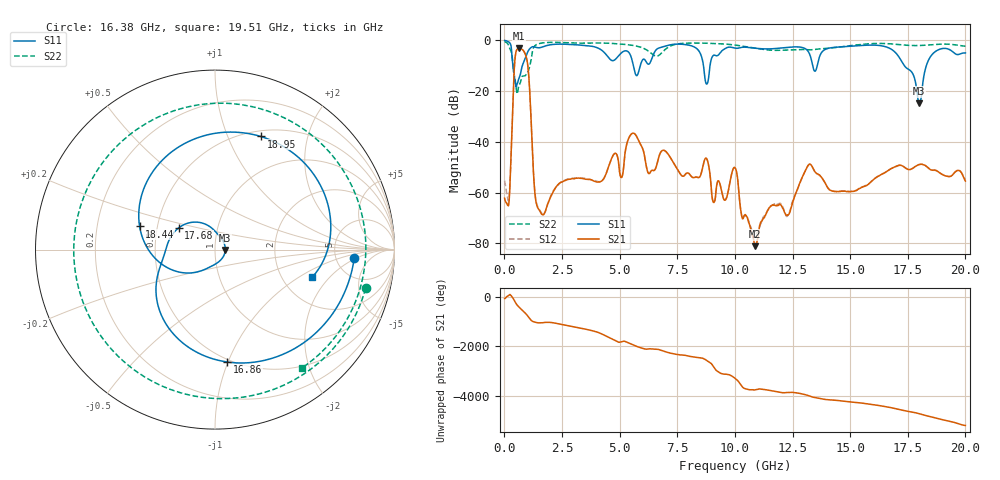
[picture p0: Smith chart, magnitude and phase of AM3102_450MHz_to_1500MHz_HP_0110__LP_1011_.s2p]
!Agilent Technologies,E8364B,MY43040894,A.07.50.67
!Agilent E8364B: A.07.50.67
!Date: Thursday, January 11, 2018 05:49:09
!Correction: S11(Full 2 Port(1,2))
!S21(Full 2 Port(1,2))
!S12(Full 2 Port(1,2))
!S22(Full 2 Port(1,2))
!S2P File: Measurements: S11, S21, S12, S22:
# Hz S  dB  R 50
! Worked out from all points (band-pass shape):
!   1601 points, 10 MHz to 20 GHz, reference 50 ohm
!   highest |S21| = -3.21 dB at 634.7 MHz (marker M1); lowest = -81.1 dB at 10.87 GHz (marker M2)
!   |S21| within 3 dB of the highest: 473.6 MHz to 934.7 MHz (461.1 MHz wide, 65.5 % of centre)
!   lowest |S11| = -24.8 dB at 18 GHz (marker M3), VSWR 1.12, Z = 56.1 - j0.257 ohm
!   |S11| at or under -10 dB: 370 MHz to 778.3 MHz (408.3 MHz wide, 71.1 % of centre); 5.594 GHz to 5.895 GHz (301.6 MHz wide, 5.25 % of centre); 17.35 GHz to 18.31 GHz (953.6 MHz wide, 5.35 % of centre)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
!   |S22| runs from -21.1 to -0.5 dB; largest |S21 - S12| = 0.0035
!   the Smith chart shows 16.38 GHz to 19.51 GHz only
!   S11 on the Smith chart (normalised r, x): 16.38 GHz: 7.52, -1.81; 16.86 GHz: 0.48, -0.99; 17.68 GHz: 0.65, +0.17; 18.44 GHz: 0.40, +0.13; 18.95 GHz: 0.56, +1.32; 19.51 GHz: 2.92, -1.32
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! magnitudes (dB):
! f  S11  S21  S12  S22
! 10 MHz  -0.1  -62.2  -55.3  -0.5
! 197.4 MHz  -0.7  -64.0  -62.0  -2.4
! 447.3 MHz  -15.2  -8.7  -8.7  -14.6
! 634.7 MHz  -15.0  -3.2  -3.2  -17.9
! 997 MHz  -4.9  -8.7  -8.7  -12.7
! 1.484 GHz  -3.0  -66.5  -66.1  -1.4
! 3.346 GHz  -1.9  -54.4  -54.2  -1.1
! 6.682 GHz  -3.1  -46.6  -46.6  -6.0
! 8.781 GHz  -17.3  -46.7  -46.7  -1.2
! 9.08 GHz  -5.9  -63.9  -64.0  -1.2
! 10.01 GHz  -3.1  -50.2  -50.2  -1.9
! 10.87 GHz  -3.1  -81.1  -76.7  -3.1
! 13.34 GHz  -8.6  -49.5  -49.5  -3.7
! 16.38 GHz  -2.2  -52.7  -52.7  -1.2
! 16.68 GHz  -3.0  -51.1  -51.1  -1.4
! 16.86 GHz  -4.0  -50.1  -50.1  -1.5
! 17.68 GHz  -12.6  -50.6  -50.6  -2.1
! 18 GHz  -24.8  -48.9  -48.9  -2.1
! 18.44 GHz  -7.1  -50.7  -50.6  -1.8
! 18.95 GHz  -3.3  -52.6  -52.6  -1.5
! 19.51 GHz  -5.0  -52.3  -52.3  -1.7
! 20 GHz  -5.0  -55.4  -54.9  -2.3
